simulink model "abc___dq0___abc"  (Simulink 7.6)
settings: Solver=FixedStepDiscrete  StartTime=0.0  StopTime=6/f  FixedStep=Ts  RelTol=1e-3
InitFcn:
  | f=60;
  | Ts=2e-5;
  | clc
  | close all
libraries: powerlib_extras x3

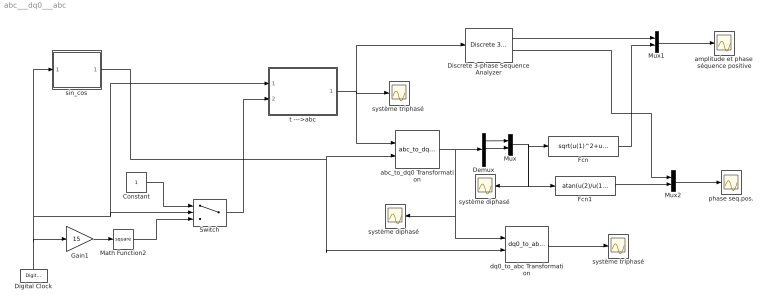
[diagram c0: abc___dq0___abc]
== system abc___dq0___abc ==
  Constant : Constant
  Demux : Demux  Outputs=3
  Digital Clock : DigitalClock  SampleTime=Ts
  Discrete 3-phase Sequence Analyzer : powerlib_extras/Discrete Measurements/Discrete 3-phase Sequence Analyzer  DialogController=POWERSYS.PowerSysDialog  SystemSampleTime=-1  Freq=60  n=1  seq=Positive  Par_Init=[1.5 0.5]  Ts=Ts
  Fcn : Fcn  Expr=sqrt(u(1)^2+u(2)^2)
  Fcn1 : Fcn  Expr=atan(u(2)/u(1))
  Gain1 : Gain  Gain=15
  Math Function2 : Math  Operator=square
  Mux : Mux  Inputs=2
  Mux1 : Mux  Inputs=2
  Mux2 : Mux  Inputs=2
  Switch : Switch  Threshold=3/f  SampleTime=Ts
  abc_to_dq0 Transformation : powerlib_extras/Measurements/abc_to_dq0 Transformation  DialogController=POWERSYS.PowerSysDialog  SystemSampleTime=-1
  amplitude et phase  séquence positive : Scope
  dq0_to_abc Transformation : powerlib_extras/Measurements/dq0_to_abc Transformation  DialogController=POWERSYS.PowerSysDialog  SystemSampleTime=-1
  phase seq.pos. : Scope
  sin_cos : Subsystem
  "système diphasé " : Scope
  "système diphasé  " : Scope
  système triphasé : Scope
  "système triphasé " : Scope
  t --->abc : Subsystem
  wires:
  t --->abc/1(abc) -> abc_to_dq0 Transformation/1, Discrete 3-phase Sequence Analyzer/1, "système triphasé "/1
  sin_cos/1(sin_cos) -> abc_to_dq0 Transformation/2, dq0_to_abc Transformation/2
  dq0_to_abc Transformation/1 -> système triphasé/1
  abc_to_dq0 Transformation/1 -> Demux/1, dq0_to_abc Transformation/1, "système diphasé  "/1
  Demux/1 -> Mux/1
  Mux/1 -> Fcn/1, Fcn1/1, "système diphasé "/1
  Gain1/1 -> Math Function2/1
  Constant/1 -> Switch/1
  Math Function2/1 -> Switch/3
  Switch/1 -> t --->abc/2(a)
  Digital Clock/1 -> Gain1/1, sin_cos/1(t), Switch/2, t --->abc/1(t)
  Demux/2 -> Mux/2
  Fcn1/1 -> Mux2/2
  Mux1/1 -> amplitude et phase  séquence positive/1
  Discrete 3-phase Sequence Analyzer/1 -> Mux1/1
  Fcn/1 -> Mux1/2
  Discrete 3-phase Sequence Analyzer/2 -> Mux2/1
  Mux2/1 -> phase seq.pos./1

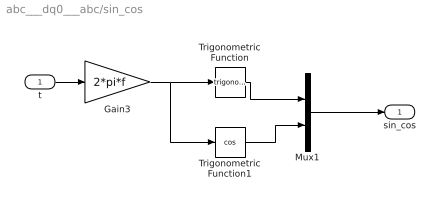
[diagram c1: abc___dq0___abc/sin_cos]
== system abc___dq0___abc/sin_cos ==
  t : Inport
  Gain3 : Gain  Gain=2*pi*f
  Mux1 : Mux  Inputs=2
  Trigonometric Function : Trigonometry
  Trigonometric Function1 : Trigonometry  Operator=cos
  sin_cos : Outport
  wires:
  Gain3/1 -> Trigonometric Function/1, Trigonometric Function1/1
  Trigonometric Function/1 -> Mux1/1
  Trigonometric Function1/1 -> Mux1/2
  t/1 -> Gain3/1
  Mux1/1 -> sin_cos/1

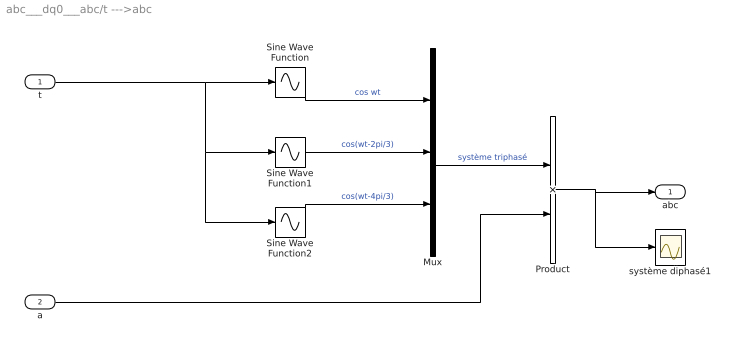
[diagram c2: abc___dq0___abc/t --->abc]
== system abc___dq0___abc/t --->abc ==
  t : Inport
  a : Inport  Port=2
  Mux : Mux  Inputs=3
  Product : Product
  Sine Wave Function : Sin  TimeSource=Use external signal  Frequency=2*pi*f  SampleTime=0
  Sine Wave Function1 : Sin  TimeSource=Use external signal  Frequency=2*pi*f  Phase=-2*pi/3  SampleTime=0
  Sine Wave Function2 : Sin  TimeSource=Use external signal  Frequency=2*pi*f  Phase=-4*pi/3  SampleTime=0
  système diphasé1 : Scope
  abc : Outport
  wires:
  Sine Wave Function1/1 -> Mux/2  "cos(wt-2pi/3)"
  Sine Wave Function/1 -> Mux/1  "cos wt"
  Sine Wave Function2/1 -> Mux/3  "cos(wt-4pi/3)"
  t/1 -> Sine Wave Function/1, Sine Wave Function1/1, Sine Wave Function2/1
  Mux/1 -> Product/1  "système triphasé"
  Product/1 -> abc/1, système diphasé1/1
  a/1 -> Product/2
